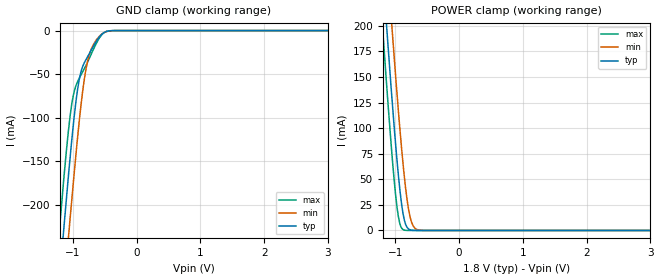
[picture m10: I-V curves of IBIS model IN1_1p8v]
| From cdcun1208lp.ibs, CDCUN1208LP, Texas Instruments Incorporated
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[Model]   IN1_1p8v
Model_type   Input
Vinl = 0.7
Vinh = 1.28
|   typ   min   max
C_comp   9.3816pF   8.2418pF   10.6638pF
[Voltage Range]   1.8   1.7   1.9
[Temperature Range]   27   105   -40
[Power Clamp Reference]   1.8   1.7   1.9
[GND Clamp Reference]   -0   0   -0
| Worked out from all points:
|   GND clamp passes 1 mA (typ) near -0.47 V on its own axis
|   POWER clamp passes 1 mA (typ) near -0.78 V on its own axis
[GND Clamp]
|   Voltage   I(typ)   I(min)   I(max)
-1.8V     -826.4mA   -895.1mA   -771.8mA
-1.214V   -289.2mA   -359.7mA   -231.4mA
-1.143V   -228.1mA   -298.8mA   -170.5mA
-1.067V   -164.4mA   -235.3mA   -113.1mA
-995.6mV  -110mA     -176.7mA   -75.14mA
-925.6mV  -67.11mA   -122.2mA   -58.6mA
-859.2mV  -43.85mA   -77.2mA    -48.98mA
-792.5mV  -33.06mA   -43.22mA   -39.74mA
-748.6mV  -27.26mA   -29.06mA   -32.84mA
-679.3mV  -18.06mA   -16.25mA   -21.73mA
-510.9mV  -2.198mA   -2.339mA   -2.38mA
3.595V    0A         0A         0A
[POWER Clamp]
|   Voltage   I(typ)   I(min)   I(max)
-1.8V     821.7mA    891.7mA    766.5mA
-1.207V   261.3mA    333.2mA    203.7mA
-1.13V    192.9mA    264.4mA    136mA
-1.045V   121.4mA    190.5mA    67.16mA
-995.6mV  83.54mA    150.3mA    34.11mA
-954.4mV  54.7mA     117.9mA    13.87mA
-868.1mV  12.74mA    57.5mA     522.1uA
-816.1mV  2.993mA    29.66mA    57.65uA
-770.2mV  657.4uA    13.3mA     17.19uA
-704.1mV  63.87uA    2.917mA    13.11uA
-627.8mV  9.844uA    370.3uA    13.03uA
3.595V    0A         0A         0A
